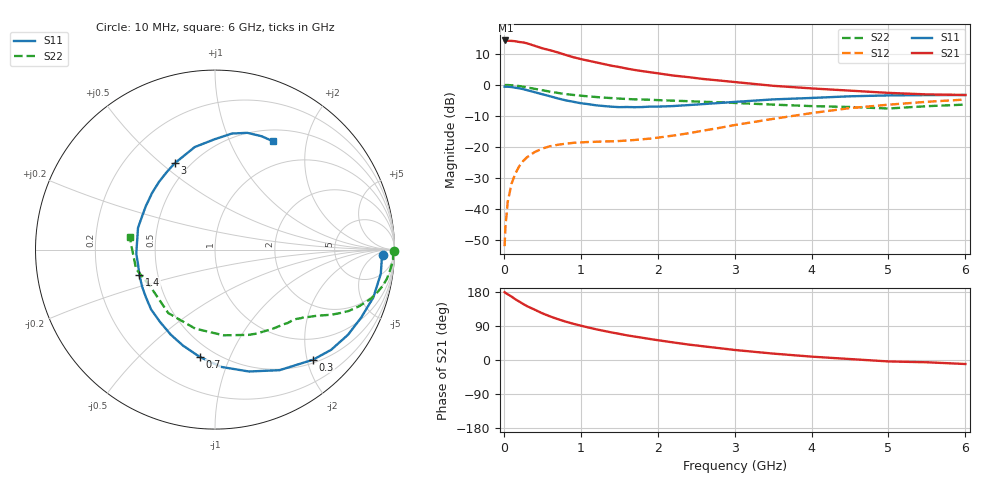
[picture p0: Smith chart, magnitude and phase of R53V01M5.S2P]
! SIEMENS Small Signal Semiconductors
! BFR183
! Si NPN RF Bipolar Junction Transistor in SOT23
! VCE = 3 V  IC = 1.5 mA
! Common Emitter S-Parameters:  May  1996
# GHz  S  MA  R  50
!  f  S11  S21  S12  S22
! GHz  MAG  ANG  MAG  ANG  MAG  ANG  MAG  ANG
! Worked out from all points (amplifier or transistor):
!   36 points, 10 MHz to 6 GHz, reference 50 ohm
!   highest |S21| = 14.3 dB at 20 MHz (marker M1)
!   |S21| within 3 dB of that: start of sweep to 575.6 MHz
!   unconditionally stable (mu >= 1): 1.496 GHz to 2.863 GHz
!   at 250 MHz: K = 0.19, MSG = 19.1 dB, |S12| = -24.6 dB
!   at 1.4 GHz: K = 0.95, MSG = 12.2 dB, |S12| = -18.2 dB
!   at 6 GHz: K = 0.93, MSG = 0.7 dB, |S12| = -4.7 dB
!   S11 on the Smith chart (normalised r, x): 10 MHz: 24, -11; 300 MHz: 0.56, -2.11; 700 MHz: 0.41, -0.78; 1.4 GHz: 0.39, -0.14; 3 GHz: 0.41, +0.55; 6 GHz: 0.65, +1.47
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0.01  0.9351 -1.8  5.134 179.1  0.0025 85.7  0.9982 -0.6
0.02  0.9308 -3.3  5.198 177.3  0.005 87.4  0.9926 -1.3
0.05  0.9335 -8.3  5.143 173.6  0.0129 84.5  0.9935 -3.3
0.1  0.9216 -16.8  5.114 167.4  0.0254 81.2  0.9835 -6.4
0.15  0.8983 -24.9  5.049 160.2  0.0372 75.4  0.9717 -9.6
0.25  0.8546 -40.8  4.832 148.0  0.0588 67.2  0.934 -14.9
0.3  0.8215 -48.3  4.68 142.2  0.0677 63.2  0.9103 -17.5
0.4  0.7622 -61.8  4.265 132.9  0.0823 56.4  0.8623 -21.5
0.5  0.7052 -74.4  3.882 123.2  0.0938 51.3  0.819 -24.7
0.6  0.6546 -86.9  3.617 115.1  0.1022 46.9  0.7767 -27.2
0.7  0.6045 -98.0  3.338 108.0  0.1079 43.6  0.7417 -29.3
0.8  0.5635 -108.5  3.048 101.5  0.1123 40.9  0.71 -31.0
0.9  0.5338 -117.6  2.797 95.8  0.1159 39.3  0.6873 -32.3
1.1  0.4877 -136.9  2.449 85.8  0.1197 37.4  0.6514 -35.0
1.4  0.4441 -161.5  2.035 72.7  0.1226 38.1  0.6116 -38.7
1.8  0.4383 170.4  1.665 58.7  0.1325 43.5  0.5803 -43.7
2.2  0.4547 148.2  1.413 46.4  0.1518 50.1  0.5555 -50.4
3  0.5306 115.1  1.11 26.5  0.2246 54.9  0.5104 -68.6
3.5  0.5823 101.2  0.965 16.9  0.2824 52.3  0.4798 -84.3
4.5  0.6535 81.7  0.806 2.5  0.4217 40.2  0.4391 -126.3
5.5  0.6829 67.7  0.701 -6.0  0.5327 24.5  0.4526 -166.2
6  0.6848 61.8  0.686 -10.6  0.5789 15.0  0.4803 171.8
